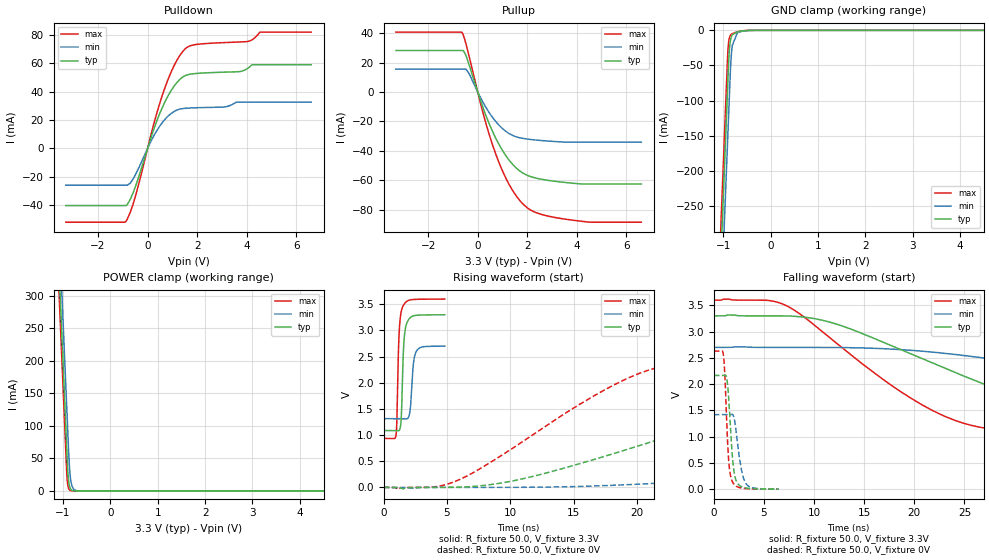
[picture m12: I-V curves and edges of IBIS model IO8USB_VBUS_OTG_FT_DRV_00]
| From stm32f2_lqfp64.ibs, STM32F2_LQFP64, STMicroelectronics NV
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| *** New cell (Generated with 5.14beta1 (Sep 20 2010 13:23:23))
[Model]   IO8USB_VBUS_OTG_FT_DRV_00
Model_type 3-state
Polarity   Non-Inverting
Enable   Active-Low
| CAP_THRESHOLD on pad IOV33 is "CMOS" :
| Rising=10.0% of vddio   Falling=90.0% of vddio
| C_comp min and max val. don't necessarily correlate with the min and max pvt
| but are the smallest and greatest pad capacitance found.
| var   typ   min   max
C_comp   2.70355pF  2.58515pF  2.87895pF
Vmeas = 1.65V   | Reference voltage for timing measurements
Cref  = 50.0pF   | Timing specification test load capacitance value
Rref  = 10.0MOhm   | Timing specification test load resistance value
Vref  = 1.65V   | Timing specification test load voltage
[Model Spec]
| variable   typ   min   max
[Temperature Range] 25.0 125.0 -40.0
| variable   typ   min   max
[Voltage Range] 3.3V 2.7V 3.6V
| variable   typ   min   max
[POWER Clamp Reference] 3.3V 2.7V 3.6V
| variable   typ   min   max
[GND Clamp Reference] 0V 0V 0V
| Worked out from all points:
|   slope of the pulldown table from 0 to 0.495 V, typ, clamps not added: 20 ohm
|   slope of the pullup table from 0 to 0.495 V, typ, clamps not added: 21.7 ohm
|   GND clamp passes 1 mA (typ) near -0.61 V on its own axis
|   POWER clamp passes 1 mA (typ) near -0.81 V on its own axis
|   rising waveform, R_fixture 50.0, V_fixture 3.3V: 20-80 % time 202ps typ, 245ps min, 188ps max; typ from 1.09 V to 3.3 V
|   falling waveform, R_fixture 50.0, V_fixture 3.3V: 20-80 % time 18.1ns typ, 35.4ns min, 11.7ns max; typ from 3.3 V to 1.09 V
|   rising waveform, R_fixture 50.0, V_fixture 0V: 20-80 % time 19.1ns typ, 43.3ns min, 10.7ns max; typ from 0 V to 2.17 V
|   falling waveform, R_fixture 50.0, V_fixture 0V: 20-80 % time 463ps typ, 655ps min, 372ps max; typ from 2.17 V to 0 V
[POWER Clamp]
-3.3V     4.11A      4.173A     4.072A
-1.09V    352.5mA    415.9mA    314.5mA
-1.05V    284.5mA    347.9mA    246.5mA
-1.01V    216.5mA    279.9mA    178.5mA
-920mV    63.51mA    126.9mA    25.85mA
-900mV    31.51mA    92.9mA     9.552mA
-890mV    21.35mA    75.9mA     5.807mA
-870mV    9.804mA    44.01mA    2.146mA
-840mV    3.05mA     18.36mA    482.1uA
-780mV    295.2uA    3.193mA    24.34uA
-660mV    2.764uA    96.47uA    62.42nA
6.6V      0A         0A         0A
[GND Clamp]
-3.3V     -4.149A    -4.224A    -4.103A
-1.06V    -341.2mA   -416.1mA   -295.1mA
-940mV    -137.2mA   -212.1mA   -91.08mA
-910mV    -86.19mA   -161.1mA   -40.08mA
-900mV    -69.19mA   -144.1mA   -27.04mA
-880mV    -37.32mA   -110.1mA   -13.88mA
-860mV    -20.03mA   -76.14mA   -8.588mA
-840mV    -11.71mA   -45.57mA   -6.266mA
-810mV    -6.348mA   -21.68mA   -4.67mA
-700mV    -2.155mA   -3.174mA   -2.051mA
-470mV    -142.2uA   -334.3uA   -67.55uA
6.6V      13.96nA    1.746uA    94.44pA
| variable   typ   min   max
[Pullup Reference] 3.3V 2.7V 3.6V
| variable   typ   min   max
[Pulldown Reference] 0V 0V 0V
[Pullup]
-3.3V     28.27mA    15.58mA    40.81mA
-630mV    28.27mA    15.58mA    40.39mA
-480mV    25.11mA    15.58mA    33.22mA
-350mV    18.69mA    12.64mA    24.51mA
240mV     -11.89mA   -7.822mA   -15.87mA
710mV     -30.8mA    -19.68mA   -41.36mA
1.3V      -47.02mA   -28.56mA   -63.9mA
1.65V     -53.05mA   -30.92mA   -72.82mA
2.01V     -56.71mA   -31.98mA   -78.86mA
2.7V      -59.67mA   -33.14mA   -83.8mA
4.01V     -62.27mA   -34.07mA   -87.53mA
6.6V      -62.54mA   -34.07mA   -88.51mA
[Pulldown]
-3.3V     -40.26mA   -25.94mA   -51.99mA
-870mV    -40.25mA   -25.94mA   -51.33mA
-700mV    -35.92mA   -24.51mA   -45.06mA
-470mV    -25.89mA   -17.87mA   -32.39mA
240mV     12.97mA    8.52mA     16.62mA
590mV     28.62mA    18.11mA    37.2mA
1.07V     43.85mA    26mA       58.31mA
1.54V     51.42mA    28.24mA    70.48mA
2.01V     52.82mA    28.63mA    73.27mA
4.01V     56.01mA    32.56mA    75.18mA
4.53V     58.89mA    32.56mA    81.88mA
6.6V      58.89mA    32.56mA    81.88mA
[Ramp]
dV/dt_r 1.29886V/19.12357ns 851.12644mV/43.33795ns 1.57728V/10.68315ns
dV/dt_f 1.3278V/18.11658ns 831.26226mV/35.41776ns 1.59819V/11.72409ns
R_load = 50.0
| Removed startup time: 0s 0s 0s  .
| Removed end time: 4.822ns.
[Rising Waveform]
R_fixture   = 50.0
V_fixture   = 3.3V
V_fixture_min = 2.7V
V_fixture_max = 3.6V
0s        1.087V     1.314V     936.3mV
976ps     1.087V     1.314V     999mV
1.04ns    1.086V     1.314V     1.259V
1.224ns   1.09V      1.314V     2.961V
1.38ns    1.291V     1.314V     3.351V
1.498ns   2.169V     1.314V     3.45V
1.658ns   2.939V     1.312V     3.514V
1.988ns   3.214V     1.356V     3.575V
2.56ns    3.288V     2.592V     3.594V
4.826ns   3.299V     2.699V     3.599V
| Removed startup time: 0s 0s 0s  .
| Removed end time: 250.44ns.
[Falling Waveform]
R_fixture   = 50.0
V_fixture   = 3.3V
V_fixture_min = 2.7V
V_fixture_max = 3.6V
0s        3.3V       2.7V       3.6V
6.6ns     3.3V       2.7V       3.546V
11.56ns   3.182V     2.7V       2.886V
18.04ns   2.708V     2.665V     1.935V
23ns      2.308V     2.588V     1.391V
33.52ns   1.567V     2.326V     1.047V
47.8ns    1.228V     1.932V     971.7mV
63.44ns   1.145V     1.615V     948.9mV
84.76ns   1.107V     1.445V     940mV
250.5ns   1.087V     1.315V     936.3mV
| Removed startup time: 0s 0s 0s  .
| Removed end time: 242.2ns.
[Rising Waveform]
R_fixture   = 50.0
V_fixture   = 0V
V_fixture_min = 0V
V_fixture_max = 0V
0s        10.11nV    410.7nV    7.11nV
6.08ns    5.428mV    -154.2uV   160.1mV
11.36ns   185.5mV    2.912mV    937.4mV
20.52ns   824mV      66.3mV     2.209V
30.68ns   1.53V      236.9mV    2.542V
37.6ns    1.863V     382.3mV    2.592V
48.36ns   2.049V     628.5mV    2.618V
69.12ns   2.14V      1.038V     2.627V
94.12ns   2.16V      1.289V     2.629V
242.3ns   2.165V     1.419V     2.629V
| Removed startup time: 0s 0s 0s  .
| Removed end time: 6.462ns.
[Falling Waveform]
R_fixture   = 50.0
V_fixture   = 0V
V_fixture_min = 0V
V_fixture_max = 0V
0s        2.165V     1.419V     2.629V
954ps     2.165V     1.419V     2.563V
1.136ns   2.171V     1.419V     2.052V
1.264ns   2.137V     1.418V     1.404V
1.472ns   1.782V     1.419V     582.2mV
1.85ns    637.6mV    1.426V     145.2mV
2.244ns   158.1mV    1.077V     56.38mV
2.73ns    51.01mV    403.3mV    24.09mV
3.2ns     22.94mV    107.3mV    11.98mV
6.466ns   492.2uV    518.5uV    630.8uV
